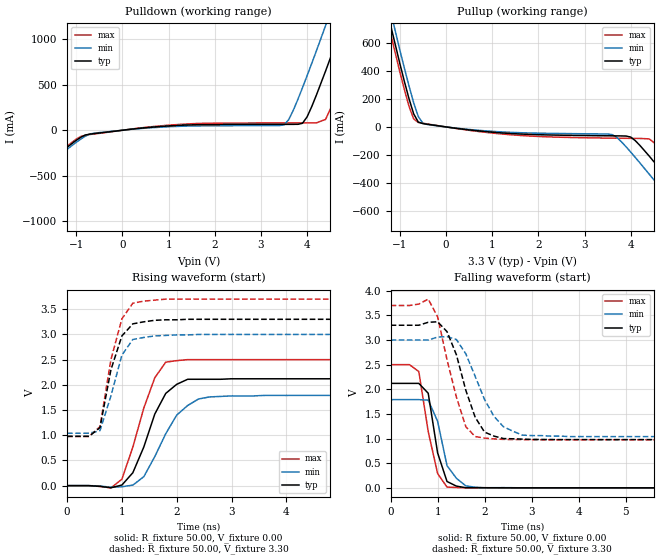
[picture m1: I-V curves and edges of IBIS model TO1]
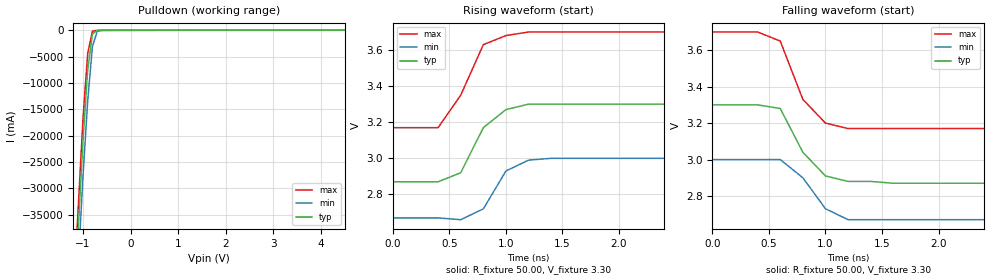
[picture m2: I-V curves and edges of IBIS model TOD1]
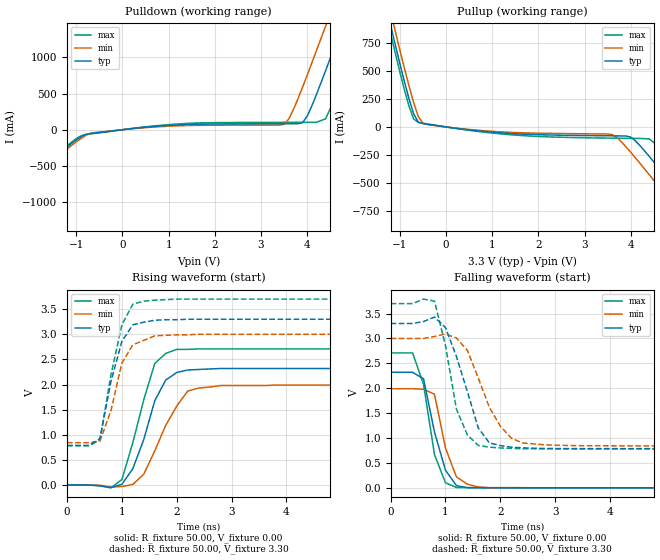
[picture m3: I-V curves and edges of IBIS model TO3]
|   * 950211af.ibs * IBIS 2.1 Model for ICS950211AF
| Rev History
| Rev No.   Description
| 1.0   Initial release with Updated Parasitic Parameters
[IBIS Ver]   2.1
[File name]   950211f.ibs
[Date]   August 6, 2001
[File Rev]   1.0
[Source]   Originated at Integrated Circuit Systems, Inc.
[Disclaimer]
(C) Copyright Integrated Circuit Systems, Inc. 1997
   All rights reserved
ICS hereby grants the user of this 950211 IBIS model a non-exclusive,
nontransferable license to use this IBIS model under the following terms.
Before using this IBIS model, the user should read this license.
If the user does not accept these terms,  the IBIS model should be
returned to ICS within 30 days.
   The user is granted this license only to use the IBIS model and
is not granted rights to sell, load, rent, lease or license the IBIS
model in whole or in part, or in modified form to anyone other than
user. User may modify the IBIS model to suit its specific
applications but rights to derivative works and such modifications
shall belong to ICS.
   This IBIS model is provided on an "AS IS" basis and ICS makes
absolutely no warranty with respect to the information contained
herein. ICS DISCLAIMS AND CUSTOMER WAIVES ALL WARRANTIES, EXPRESS
OR IMPLIED, INCLUDING WARRANTIES OF MERCHANTABILITY OR FITNESS FOR
A PARTICULAR PURPOSE. The entire risk as to quality and performance
is with the Customer. ACCORDINGLY, IN NO EVENT SHALL THE COMPANY BE
LIABLE FOR ANY DAMAGES, WHETHER IN CONTRACT OR TORT,INCLUDING ANY
LOST PROFITS OR OTHER INCIDENTAL, CONSEQUENTIAL, EXEMPLARY, OR
PUNITIVE DAMAGES ARISING OUT OF THE USE OR APPLICATION OF THE IBIS
model provided in this package. Further, ICS reserves the right to
make changes without notice to any product herein to improve
reliability, function, or design. ICS does not convey any license
under patent rights or any other intellectual property rights,
including those of third parties.
   ICS is not obligated to provide maintenance or support
for the licensed IBIS model.
|   COMPONENT: 950211AF
[Component]   950211AF
[Manufacturer]  ICS
[Package]
|variable   typ   min   max
R_pkg   81.1m   62.2m   100.0m
L_pkg   6.7nH   4.9nH   8.5nH
C_pkg   0.53pF  0.21pF  0.85pF
[Pin]   signal_name   model_name   R_pin   L_pin   C_pin
  1   VDDREF   POWER
  2   X1   TI9
  3   X2   TO7
  4   VSS   GND
  5   PCI_FS0   TIO8
  6   PCI_FS1   TIO8
  7   PCI_FS2   TIO8
  8   VDDPCI   POWER
  9   VSS   GND
  10   PCI_ENWD   TIO8
  11   PCI1   TO1
  12   PCI2   TO1
  13   PCI3   TO1
  14   VDDPCI   POWER
  15   VSS   GND
  16   PCI4   TO1
  17   PCI5   TO1
  18   PCI6   TO1
  19   VDD66   POWER
  20   VSS   GND
  21   3V66_2   TO3
  22   3V66_3   TO3
  23   3V66_4   TO3
  24   3V66_5   TO3
  25   PDB   TI13
  26   VDDA   POWER
  27   VSS   GND
  28   PWRGDB   TI13
  29   SDA   TOD1
  30   SCL   TI11
  31   VSS   GND
  32   VDD66   POWER
  33   3V66_0   TIO1
  34   PCISTB   TI7
  35   3V66_1_VCH   TO3
  36   VSS   GND
  37   VDD48   POWER
  38   48MHZ_DOT   TO1
  39   48_FS3   TIO1
  40   FS2   TI7
  41   VSS   GND
  42   IREF   TI7
  43   MULT_SEL0   TI13
  44   CPUC2   THB3
  45   CPUT2   TH3
  46   VDDCPU   POWER
  47   VSS   GND
  48   CPUC1   THB3
  49   CPUT1   TH3
  50   VDDCPU   POWER
  51   CPUC0   THB3
  52   CPUT0   TH3
  53   CPUSTPB   TI7
  54   FS0   TI7
  55   FS1   TI7
  56   REF   TIO1
| Models and submodels in the file (13): TO1 (Output), TOD1 (Open_drain), TO3 (Output), TO5 (Open_drain), TO7 (Output), TI9 (Input), TI7 (Input), TI11 (Input), TIO8 (I/O), TI13 (Input), TH3 (Open_source), THB3 (Open_source), TIO1 (I/O)
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|   Model TO1
[Model]   TO1
Model_type   Output
Polarity   Non-Inverting
C_comp   5.50pF   5.00pF   6.00pF
[Temperature Range]   27.00   70.00   0.00
[Voltage Range]   3.30V   3.00V   3.70V
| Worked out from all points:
|   slope of the pulldown table from 0 to 0.495 V, typ, clamps not added: 18.1 ohm
|   slope of the pullup table from 0 to 0.495 V, typ, clamps not added: 23.6 ohm
|   rising waveform, R_fixture 50.00, V_fixture 0.00: 20-80 % time 469ps typ, 543ps min, 437ps max; typ from 0 V to 2.12 V
|   rising waveform, R_fixture 50.00, V_fixture 3.30: 20-80 % time 309ps typ, 312ps min, 309ps max; typ from 0.978 V to 3.3 V
|   falling waveform, R_fixture 50.00, V_fixture 0.00: 20-80 % time 261ps typ, 309ps min, 291ps max; typ from 2.12 V to 0 V
|   falling waveform, R_fixture 50.00, V_fixture 3.30: 20-80 % time 453ps typ, 568ps min, 434ps max; typ from 3.3 V to 0.978 V
[Pulldown]
| voltage   I(typ)   I(min)   I(max)
-3.3V     -1.04A     -1.06A     -1.02A
-1V       -109.9mA   -132.1mA   -97.14mA
-700mV    -42.1mA    -41.03mA   -46.68mA
1.3V      55.25mA    44.2mA     65.96mA
3.5V      64.71mA    59.32mA    80.34mA
3.6V      64.79mA    115.3mA    80.43mA
3.9V      76.61mA    467.8mA    80.69mA
4.1V      259.7mA    735mA      80.89mA
4.4V      651.1mA    1.15A      119mA
4.8V      1.2A       1.71A      606.8mA
5.2V      1.77A      2.27A      1.16A
6.2V      3.2A       3.71A      2.59A
[Pullup]
| voltage   I(typ)   I(min)   I(max)
-3.3V     3.69A      3.78A      3.63A
-1.5V     1.14A      1.24A      1.08A
-1V       453.7mA    550.5mA    393.6mA
-800mV    199.9mA    291.4mA    145.9mA
-600mV    34.46mA    74.11mA    32.02mA
500mV     -21.21mA   -18.05mA   -24.27mA
3.6V      -63.88mA   -55.08mA   -80.45mA
4V        -72.8mA    -180mA     -81.92mA
4.4V      -208.3mA   -337.9mA   -85.64mA
5.4V      -613.2mA   -746.2mA   -452.7mA
5.6V      -695.6mA   -828.6mA   -534.6mA
6.2V      -943.4mA   -1.08A     -781.9mA
[Ramp]
| variable   typ   min   max
dV/dt_r   1.27/409.06p   1.07/515.73p   1.50/360.46p
dV/dt_f   1.39/400.00p   1.18/500.00p   1.63/400.00p
[Rising Waveform]
R_fixture = 50.00
V_fixture = 0.00
V_fixture_min = 0.00
V_fixture_max = 0.00
| time   V(typ)   V(min)   V(max)
0s        0V         0V         0V
800ps     -41.54mV   -33.17mV   -43.75mV
1ns       11.98mV    -21.22mV   127.4mV
1.2ns     256.8mV    10.82mV    765.3mV
1.4ns     767.5mV    177.9mV    1.54V
1.6ns     1.42V      576.3mV    2.14V
1.8ns     1.83V      1.03V      2.45V
2.2ns     2.11V      1.59V      2.5V
2.6ns     2.11V      1.76V      2.5V
10ns      2.12V      1.79V      2.5V
[Rising Waveform]
R_fixture = 50.00
V_fixture = 3.30
V_fixture_min = 3.00
V_fixture_max = 3.70
| time   V(typ)   V(min)   V(max)
0s        978.2mV    1.04V      976.3mV
400ps     978.3mV    1.04V      976.4mV
600ps     1.15V      1.09V      1.17V
800ps     2.3V       1.78V      2.5V
1ns       2.97V      2.59V      3.31V
1.2ns     3.21V      2.9V       3.62V
1.6ns     3.28V      2.97V      3.68V
1.8ns     3.29V      2.98V      3.7V
2.4ns     3.3V       3V         3.7V
10ns      3.3V       3V         3.7V
[Falling Waveform]
R_fixture = 50.00
V_fixture = 0.00
V_fixture_min = 0.00
V_fixture_max = 0.00
| time   V(typ)   V(min)   V(max)
0s        2.12V      1.79V      2.5V
400ps     2.12V      1.79V      2.5V
600ps     2.12V      1.79V      2.36V
800ps     1.92V      1.78V      1.14V
1ns       707.9mV    1.35V      288.9mV
1.2ns     128.5mV    449.5mV    14.94mV
1.4ns     34.65mV    193.1mV    6.63mV
1.6ns     1.64mV     39.61mV    1.42mV
2ns       2.08mV     534.9uV    1.66mV
10ns      -2.48uV    3.8uV      3.88uV
[Falling Waveform]
R_fixture = 50.00
V_fixture = 3.30
V_fixture_min = 3.00
V_fixture_max = 3.70
| time   V(typ)   V(min)   V(max)
0s        3.3V       3V         3.7V
800ps     3.36V      3V         3.83V
1ns       3.37V      3.06V      3.47V
1.2ns     3.17V      3.07V      2.6V
1.4ns     2.7V       3.01V      1.84V
1.6ns     1.98V      2.72V      1.24V
1.8ns     1.43V      2.26V      1.04V
2.2ns     1.05V      1.45V      992.8mV
2.8ns     988.1mV    1.07V      978.2mV
10ns      978.2mV    1.04V      976.3mV
|   Model TOD1
[Model]   TOD1
Model_type   Open_drain
Polarity   Inverting
C_comp   5.50pF   5.00pF   6.00pF
[Temperature Range]   27.00   70.00   0.00
[Voltage Range]   3.30V   3.00V   3.70V
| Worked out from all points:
|   slope of the pulldown table from 0 to 0.495 V, typ, clamps not added: 122 ohm
|   rising waveform, R_fixture 50.00, V_fixture 3.30: 20-80 % time 259ps typ, 198ps min, 257ps max; typ from 2.87 V to 3.3 V
|   falling waveform, R_fixture 50.00, V_fixture 3.30: 20-80 % time 274ps typ, 261ps min, 248ps max; typ from 3.3 V to 2.87 V
[Pulldown]
| voltage   I(typ)   I(min)   I(max)
-3.3V     -431.7A    -437.9A    -427.9A
-1.5V     -105.8A    -112.6A    -101.5A
-1V       -21.13A    -27.91A    -16.98A
-900mV    -7.57A     -13.43A    -4.4A
-800mV    -689.4mA   -3.07A     -180.9mA
-700mV    -25mA      -186.7mA   -11.64mA
-600mV    -6.45mA    -11.8mA    -6.72mA
6.2V      12.17mA    9.78mA     14.58mA
[Ramp]
| variable   typ   min   max
dV/dt_r   255.60m/191.81p   201.00m/183.01p   319.20m/189.70p
dV/dt_f   255.60m/100.00p   201.00m/200.00p   319.20m/200.00p
[Rising Waveform]
R_fixture = 50.00
V_fixture = 3.30
V_fixture_min = 3.00
V_fixture_max = 3.70
| time   V(typ)   V(min)   V(max)
0s        2.87V      2.67V      3.17V
400ps     2.87V      2.67V      3.17V
600ps     2.92V      2.66V      3.35V
800ps     3.17V      2.72V      3.63V
1ns       3.27V      2.93V      3.68V
1.2ns     3.3V       2.99V      3.7V
1.4ns     3.3V       3V         3.7V
10ns      3.3V       3V         3.7V
[Falling Waveform]
R_fixture = 50.00
V_fixture = 3.30
V_fixture_min = 3.00
V_fixture_max = 3.70
| time   V(typ)   V(min)   V(max)
0s        3.3V       3V         3.7V
400ps     3.3V       3V         3.7V
600ps     3.28V      3V         3.65V
800ps     3.04V      2.9V       3.33V
1ns       2.91V      2.73V      3.2V
1.2ns     2.88V      2.67V      3.17V
1.4ns     2.88V      2.67V      3.17V
1.6ns     2.87V      2.67V      3.17V
10ns      2.87V      2.67V      3.17V
|   Model TO3
[Model]   TO3
Model_type   Output
Polarity   Non-Inverting
C_comp   5.50pF   5.00pF   6.00pF
[Temperature Range]   27.00   70.00   0.00
[Voltage Range]   3.30V   3.00V   3.70V
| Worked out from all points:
|   slope of the pulldown table from 0 to 0.495 V, typ, clamps not added: 14.3 ohm
|   slope of the pullup table from 0 to 0.495 V, typ, clamps not added: 18.8 ohm
|   rising waveform, R_fixture 50.00, V_fixture 0.00: 20-80 % time 439ps typ, 537ps min, 413ps max; typ from 0 V to 2.32 V
|   rising waveform, R_fixture 50.00, V_fixture 3.30: 20-80 % time 320ps typ, 345ps min, 313ps max; typ from 0.787 V to 3.3 V
|   falling waveform, R_fixture 50.00, V_fixture 0.00: 20-80 % time 309ps typ, 285ps min, 272ps max; typ from 2.32 V to 0 V
|   falling waveform, R_fixture 50.00, V_fixture 3.30: 20-80 % time 430ps typ, 514ps min, 340ps max; typ from 3.3 V to 0.787 V
[Pulldown]
| voltage   I(typ)   I(min)   I(max)
-3.3V     -1.31A     -1.34A     -1.3A
-1V       -138.9mA   -167mA     -122.8mA
-700mV    -53.25mA   -51.89mA   -59.04mA
1.3V      69.87mA    55.91mA    83.42mA
3.5V      81.85mA    74.9mA     101.6mA
3.6V      81.95mA    144.9mA    101.7mA
3.9V      96.73mA    585.5mA    102.1mA
4.1V      325.6mA    919.5mA    102.3mA
4.4V      814.9mA    1.43A      149.9mA
4.8V      1.5A       2.13A      759.8mA
5.2V      2.21A      2.84A      1.45A
6.2V      4A         4.63A      3.24A
[Pullup]
| voltage   I(typ)   I(min)   I(max)
-3.3V     4.61A      4.72A      4.53A
-1.5V     1.42A      1.54A      1.35A
-1V       567.1mA    688.1mA    492mA
-800mV    249.9mA    364.3mA    182.4mA
-600mV    43.07mA    92.63mA    40.02mA
500mV     -26.52mA   -22.57mA   -30.33mA
3.6V      -79.85mA   -68.91mA   -100.6mA
4V        -91.11mA   -226.8mA   -102.4mA
4.4V      -262.5mA   -426.5mA   -107.1mA
5.4V      -774.5mA   -942.9mA   -571.3mA
5.6V      -878.6mA   -1.05A     -674.9mA
6.2V      -1.19A     -1.36A     -987.6mA
[Ramp]
| variable   typ   min   max
dV/dt_r   1.39/376.03p   1.19/514.85p   1.63/314.16p
dV/dt_f   1.51/400.00p   1.29/500.00p   1.75/300.00p
[Rising Waveform]
R_fixture = 50.00
V_fixture = 0.00
V_fixture_min = 0.00
V_fixture_max = 0.00
| time   V(typ)   V(min)   V(max)
0s        0V         0V         0V
800ps     -49.82mV   -38.81mV   -55.79mV
1ns       14.75mV    -29.35mV   109.4mV
1.2ns     326.9mV    12.4mV     846.8mV
1.6ns     1.68V      681.3mV    2.42V
1.8ns     2.09V      1.19V      2.62V
2ns       2.24V      1.57V      2.7V
2.2ns     2.29V      1.87V      2.7V
2.8ns     2.32V      1.98V      2.71V
10ns      2.32V      1.99V      2.71V
[Rising Waveform]
R_fixture = 50.00
V_fixture = 3.30
V_fixture_min = 3.00
V_fixture_max = 3.70
| time   V(typ)   V(min)   V(max)
0s        786.9mV    842.7mV    783.4mV
400ps     786.9mV    842.7mV    783.4mV
600ps     926.2mV    874.4mV    895.7mV
800ps     2.06V      1.48V      2.19V
1ns       2.86V      2.43V      3.19V
1.2ns     3.19V      2.79V      3.6V
1.4ns     3.24V      2.88V      3.66V
1.6ns     3.28V      2.97V      3.68V
2.4ns     3.3V       3V         3.7V
10ns      3.3V       3V         3.7V
[Falling Waveform]
R_fixture = 50.00
V_fixture = 0.00
V_fixture_min = 0.00
V_fixture_max = 0.00
| time   V(typ)   V(min)   V(max)
0s        2.32V      1.99V      2.71V
400ps     2.32V      1.99V      2.71V
600ps     2.19V      1.98V      2.08V
800ps     1.12V      1.88V      668mV
1ns       354.1mV    800.7mV    100.9mV
1.2ns     44.9mV     220.4mV    6.16mV
1.4ns     2.06mV     71.86mV    4.05mV
1.6ns     3.72mV     16.68mV    2.38mV
1.8ns     2.58mV     969.5uV    1.23mV
10ns      910nV      16.41uV    -982.1nV
[Falling Waveform]
R_fixture = 50.00
V_fixture = 3.30
V_fixture_min = 3.00
V_fixture_max = 3.70
| time   V(typ)   V(min)   V(max)
0s        3.3V       3V         3.7V
800ps     3.43V      3.04V      3.75V
1ns       3.22V      3.09V      2.86V
1.2ns     2.64V      3.01V      1.58V
1.4ns     1.93V      2.76V      1.06V
1.6ns     1.2V       2.2V       850.7mV
1.8ns     903.3mV    1.62V      817.9mV
2ns       847.6mV    1.24V      800mV
2.4ns     803.6mV    901.6mV    786mV
10ns      786.9mV    842.7mV    783.4mV
